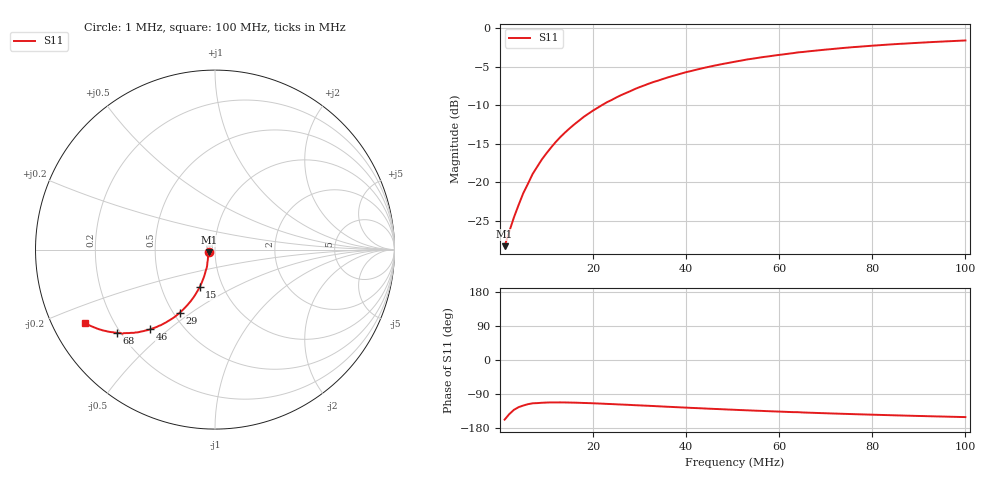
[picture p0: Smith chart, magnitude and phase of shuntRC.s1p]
# Hz S RI R 50.0
! written by SimSmith version 18.3b
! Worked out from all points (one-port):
!   100 points, 1 MHz to 100 MHz, reference 50 ohm
!   lowest |S11| = -28.3 dB at 1 MHz (marker M1), VSWR 1.08, Z = 46.6 - j1.38 ohm
!   |S11| at or under -10 dB: start of sweep to 21.9 MHz
!   S11 on the Smith chart (normalised r, x): 1 MHz: 0.93, -0.03; 15 MHz: 0.78, -0.34; 29 MHz: 0.54, -0.45; 46 MHz: 0.33, -0.43; 68 MHz: 0.19, -0.36; 100 MHz: 0.10, -0.26
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1000000  -0.0353 -0.0147
3000000  -0.039 -0.0441
4000000  -0.0401 -0.0584
5000000  -0.0425 -0.0731
7000000  -0.0463 -0.1026
9000000  -0.0546 -0.1293
1e7  -0.0584 -0.1424
1.2e7  -0.0682 -0.1693
1.4e7  -0.079 -0.1948
1.5e7  -0.0851 -0.2072
1.8e7  -0.1053 -0.2436
2e7  -0.1196 -0.2661
2.3e7  -0.1441 -0.2976
2.6e7  -0.1696 -0.3258
2.9e7  -0.1968 -0.3516
3.3e7  -0.234 -0.3816
3.9e7  -0.2924 -0.4159
4.3e7  -0.331 -0.4334
4.6e7  -0.3601 -0.4433
5.1e7  -0.4065 -0.4555
5.6e7  -0.4507 -0.4637
6.3e7  -0.5089 -0.4653
6.4e7  -0.5154 -0.4692
6.5e7  -0.5246 -0.4652
6.8e7  -0.5467 -0.4634
7.6e7  -0.6018 -0.4556
8.8e7  -0.6702 -0.4347
1e8  -0.7266 -0.4086
